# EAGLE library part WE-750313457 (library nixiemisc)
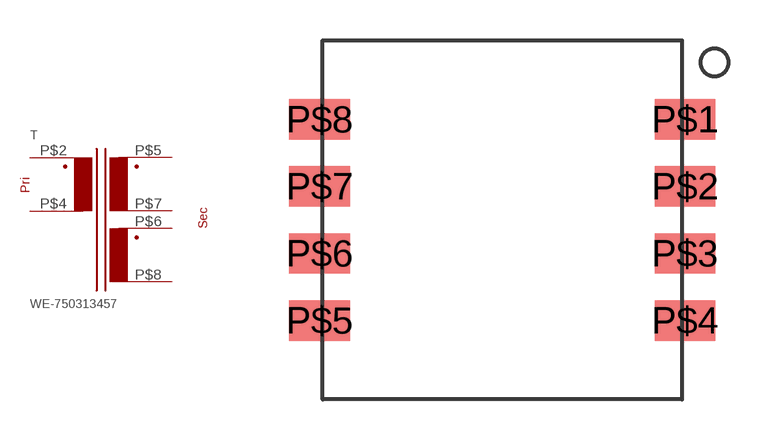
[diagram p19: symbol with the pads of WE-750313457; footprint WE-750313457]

Designator prefix T

## WE-750313457  [WE-750313457]
P$2  2  pas
P$4  4  pas
P$5  5  pas
P$6  6  pas
P$7  7  pas
P$8  8  pas

## Footprint WE-750313457 (pad centres in mm)
smd 2.25 x 1.5: P$1 6.782,3.734; P$2 6.782,1.245; P$3 6.782,-1.245; P$4 6.782,-3.734; P$5 -6.782,-3.734; P$6 -6.782,-1.245; P$7 -6.782,1.245; P$8 -6.782,3.734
